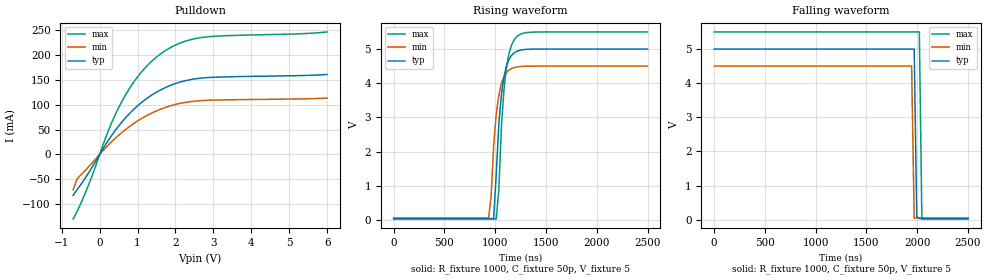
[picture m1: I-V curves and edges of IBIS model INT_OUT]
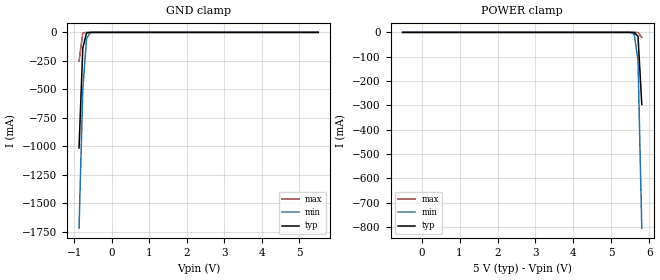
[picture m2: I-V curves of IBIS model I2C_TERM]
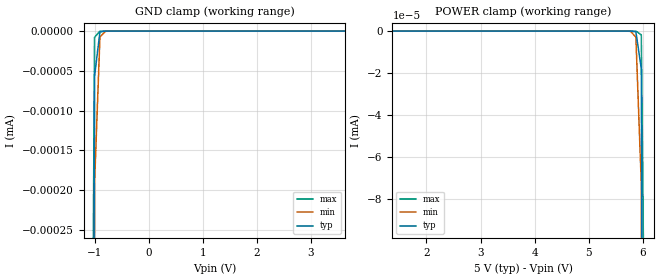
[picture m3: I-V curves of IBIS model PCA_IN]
|   NXP Semiconductors Inc.
|   Specialty Logic Products Group
|   IBIS model of PCA9545B
|   4-Channel I2C switch with
|   interrupt logic and reset
[IBIS Ver]   3.2
[Comment Char]   |_char
|  VDD Typ: 5V, Min: 4.5V, Max: 5.5V
[File name]   pca9545b_5v.ibs
[File Rev]   1.0
[Date]   Dec 05, 2007 9:30:50 AM
[Source]
Generated by Seshadri Venkataramanan with IbisToolKit at Tempe, AZ
[Notes]
[Disclaimer]
(C) Copyright 2007 NXP Semiconductors
All rights reserved
NXP Semiconductors (NXP) does not warrant that this model and any other
accompanying information (Model) accurately or fully represents the
operating characteristics and specifications of the semiconductor
products to which the Model relates.  Moreover, the Model is furnished
on an "as is" and with "all faults" basis, and without support or
warranty of any kind.  NXP disclaims all warranties, whether expressed
or implied or statutory, including without limitation all implied
warranties of non-infringement, merchantability and fitness for any
purpose, and those arising from a course of dealing or usage of trade.
NXP does not convey any license under its or any third party's patents,
copyrights or other intellectual property or proprietary rights.
You and your company assume any and all risks and liability arising out
of the application or use of the Model.
In no event shall NXP be liable for any direct, indirect, special,
consequential or incidental damages, however caused, whether in
warranty, contract or tort (including negligence), strict liability or
other legal theory, including, without limitation, for lost profits,
business interruption, or corruption or loss of data or information,
arising out of or in connection with the use of or the inability to use
the Model, even if NXP has been advised of the possibility of such
damages.
NXP provides the Model as a courtesy to our customers. You and your
company shall not distribute, convey, sell, or give the Model to anyone
else without receiving prior written permission from NXP.
NXP reserves the right to make changes without notice to the Model to
improve reliability, function, or design.
Please be aware that your receipt and subsequent use of the Model shall
serve as acceptance of these terms and conditions.  If you do not
accept these terms, return or destroy the Model immediately.
[Copyright]
2007
[Component]   PCA9545AD
Si_location Pin
Timing_location Pin
[Manufacturer]   NXP Semiconductors
[Package]
|   variable   typ   min   max
R_pkg   5.95E-02   5.36E-02   6.59E-02
L_pkg   4.21E-09   3.07E-09   5.91E-09
C_pkg   0.910E-12   0.758E-12   1.110E-12
|   SO20
[Pin] signal_name   model_name   R_pin   L_pin   C_pin
1   A0   PCA_IN   5.75E-02  5.91E-09  1.050E-12
2   A1   PCA_IN   6.25E-02  4.85E-09  1.040E-12
3   RESETB   PCA_IN   6.59E-02  3.92E-09  0.861E-12
4   INT0B   INT_IN   5.79E-02  3.32E-09  0.803E-12
5   SD0   I2C_TERM   5.36E-02  3.07E-09  0.758E-12
6   SC0   I2C_TERM   5.36E-02  3.07E-09  0.758E-12
7   INT1B   INT_IN   5.79E-02  3.32E-09  0.803E-12
8   SD1   I2C_TERM   6.59E-02  3.92E-09  0.861E-12
9   SC1   I2C_TERM   6.25E-02  4.85E-09  1.040E-12
10   Vss   GND   5.75E-02  5.91E-09  1.110E-12
11   INT2B   INT_IN   5.75E-02  5.91E-09  1.110E-12
12   SD2   I2C_TERM   6.25E-02  4.85E-09  1.040E-12
13   SC2   I2C_TERM   6.59E-02  3.92E-09  0.861E-12
14   INT3B   INT_IN   5.79E-02  3.32E-09  0.803E-12
15   SD3   I2C_TERM   5.36E-02  3.07E-09  0.758E-12
16   SC3   I2C_TERM   5.36E-02  3.07E-09  0.758E-12
17   INTB   INT_OUT   5.79E-02  3.32E-09  0.803E-12
18   SCL   I2C_TERM   6.59E-02  3.92E-09  0.861E-12
19   SDA   I2C_TERM   6.25E-02  4.85E-09  1.040E-12
20   Vdd   POWER   5.75E-02  5.91E-09  1.110E-12
[Component]   PCA9545APW
Si_location Pin
Timing_location Pin
[Manufacturer]   NXP Semiconductors
[Package]
|   variable   typ   min   max
R_pkg   7.24E-02   6.63E-02   8.34E-02
L_pkg   2.47E-09   2.09E-09   3.18E-09
C_pkg   0.341E-12   0.282E-12   0.420E-12
|   TSSOP20
[Pin] signal_name   model_name   R_pin   L_pin   C_pin
1   A0   PCA_IN   6.63E-02  3.18E-09  0.408E-12
2   A1   PCA_IN   6.67E-02  2.55E-09  0.398E-12
3   RESETB   PCA_IN   8.34E-02  2.35E-09  0.317E-12
4   INT0B   INT_IN   7.44E-02  2.16E-09  0.293E-12
5   SD0   I2C_TERM   7.10E-02  2.09E-09  0.282E-12
6   SC0   I2C_TERM   7.10E-02  2.09E-09  0.282E-12
7   INT1B   INT_IN   7.44E-02  2.16E-09  0.293E-12
8   SD1   I2C_TERM   8.34E-02  2.35E-09  0.317E-12
9   SC1   I2C_TERM   6.67E-02  2.55E-09  0.397E-12
10   Vss   GND   6.63E-02  3.18E-09  0.420E-12
11   INT2B   INT_IN   6.63E-02  3.17E-09  0.420E-12
12   SD2   I2C_TERM   6.67E-02  2.55E-09  0.397E-12
13   SC2   I2C_TERM   8.34E-02  2.35E-09  0.317E-12
14   INT3B   INT_IN   7.44E-02  2.16E-09  0.293E-12
15   SD3   I2C_TERM   7.10E-02  2.09E-09  0.282E-12
16   SC3   I2C_TERM   7.10E-02  2.09E-09  0.282E-12
17   INTB   INT_OUT   7.44E-02  2.16E-09  0.293E-12
18   SCL   I2C_TERM   8.34E-02  2.35E-09  0.317E-12
19   SDA   I2C_TERM   6.67E-02  2.55E-09  0.398E-12
20   Vdd   POWER   6.63E-02  3.17E-09  0.420E-12
[Component]   PCA9545ABS
Si_location Pin
Timing_location Pin
[Manufacturer]   NXP Semiconductors
[Package]
|   variable   typ   min   max
R_pkg   0.364   0.215   0.513
L_pkg   1.49E-09   1.04E-09   1.93E-09
C_pkg   0.149E-12   0.124E-12   0.173E-12
|   HVQFN20
[Package Model]   hvqfn20
[Pin] signal_name   model_name
1   RESETB   I2C_TERM
2   INT0B   INT_IN
3   SD0   I2C_TERM
4   SC0   I2C_TERM
5   INT1B   INT_IN
6   SD1   I2C_TERM
7   SC1   I2C_TERM
8   Vss   GND
9   INT2B   INT_IN
10   SD2   I2C_TERM
11   SC2   I2C_TERM
12   INT3B   INT_IN
13   SD3   I2C_TERM
14   SC3   I2C_TERM
15   INTB   INT_OUT
16   SCL   I2C_TERM
17   SDA   I2C_TERM
18   Vdd   POWER
19   A0   PCA_IN
20   A1   PCA_IN
[Series Pin Mapping] pin_2 model_name   function_table_group
18   6   PCA_SW   1
18   9   PCA_SW   2
18   13   PCA_SW   3
18   16   PCA_SW   4
19   5   PCA_SW   1
19   8   PCA_SW   2
19   12   PCA_SW   3
19   15   PCA_SW   4
[Series Switch Groups]
|   Function Group States
|  default
Off 1 2 3 4 /
On 1 /
On 2 /
On 3 /
On 4 /
[Define Package Model]   hvqfn20
[Manufacturer]   Unknown
[OEM]   Unknown
[Description]   none
[Number of Pins]   20
[Pin Numbers]
|   1 = RESETB
1
|   2 = INT0B
2
|   3 = SD0
3
|   4 = SC0
4
|   5 = INT1B
5
|   6 = SD1
6
|   7 = SC1
7
|   8 = VSS
8
|   9 = INT2B
9
|   10 = SD2
10
|   11 = SC2
11
|   12 = INT3B
12
|   13 = SD3
13
|   14 = SC3
14
|   15 = INTB
15
|   16 = SCL
16
|   17 = SDA
17
|   18 = VDD
18
|   19 = A0
19
|   20 = A1
20
[Model Data]
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[End Model Data]
[End Package Model]
[Model]   PCA_SW
Model_type Series_switch
C_comp   0.5p   0.5p   0.5p
[Temperature Range] 27   -40   85
[Voltage Range]   3.3   2.3   5.5
[Pullup Reference]  3.3   2.3   5.5
[Pulldown Reference]0   0   0
[On]
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[Off]
|   variable   R(typ)   R(min)   R(max)
[R Series]   1e06   1e06   1e06
|[End   PCA_SW
| [End   PCA_SW
| Models and submodels in the file (5): INT_OUT (Open_drain), I2C_TERM (Terminator), PCA_IN (Input), INT_IN (Input), PCA_SW (Series_switch)
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[Model]   INT_OUT
Model_type Open_drain
Vref=5
Vmeas=1.65
Rref=1000
Cref=1p
C_comp   2.2p   2p   2.3p
[Model Spec]
Vmeas   1.65   1.485   1.815
[Temperature Range] 27   85   -40
[Voltage Range]   5   4.5   5.5
[Pullup Reference]  5   4.5   5.5
[Pulldown Reference]0   0   0
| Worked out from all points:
|   slope of the pulldown table from 0 to 0.75 V, typ, clamps not added: 9.45 ohm
|   falling waveform, R_fixture 1000, C_fixture 50p, V_fixture 5: 20-80 % time 15.3ns typ, 15.2ns min, 15.1ns max; typ from 5 V to 0.038 V
|   rising waveform, R_fixture 1000, C_fixture 50p, V_fixture 5: 20-80 % time 73.3ns typ, 69.7ns min, 69.8ns max; typ from 0.038 V to 5 V
[Pulldown]
-700mV    -82.55mA   -71.37mA   -130.3mA
-600mV    -71.47mA   -49.68mA   -115.5mA
-300mV    -38.1mA    -25.71mA   -63.01mA
100mV     12.95mA    8.51mA     22.02mA
300mV     36.57mA    24.33mA    61.11mA
600mV     66.6mA     45.04mA    108.9mA
800mV     83.41mA    56.95mA    134.7mA
1.1V      104.4mA    72.13mA    165.9mA
1.6V      129.8mA    90.92mA    202.2mA
2.1V      145.3mA    102.5mA    223.8mA
2.7V      153.9mA    108.5mA    235.7mA
6V        161.1mA    113.4mA    246.9mA
[Falling Waveform]
R_fixture=1000
C_fixture=50p
V_fixture=5
V_fixture_min=4.5
V_fixture_max=5.5
0s        5V         4.5V       5.5V
1.944us   5V         4.5V       5.5V
1.97us    5V         52.35mV    5.5V
1.995us   96.7mV     51.74mV    5.5V
2.02us    37.66mV    51.74mV    5.5V
2.045us   37.66mV    51.74mV    22.54mV
2.5us     37.66mV    51.73mV    24.19mV
[Rising Waveform]
R_fixture=1000
C_fixture=50p
V_fixture=5
V_fixture_min=4.5
V_fixture_max=5.5
0s        37.66mV    51.74mV    24.19mV
934.3ns   37.7mV     51.77mV    24.26mV
959.6ns   37.7mV     676.9mV    24.26mV
984.8ns   37.74mV    2.18V      24.26mV
1.01us    1.341V     3.093V     24.3mV
1.035us   2.781V     3.647V     866.1mV
1.061us   3.655V     3.983V     2.692V
1.111us   4.506V     4.31V      4.47V
1.212us   4.933V     4.474V     5.362V
2.5us     5V         4.5V       5.5V
[Ramp]
R_load=1000
dV/dt_r   1.489E+0/8.641E-10   1.483E+0/1.052E-9   1.493E+0/6.606E-10
dV/dt_f   1.489E+0/3.855E-10   1.483E+0/6.984E-10   1.493E+0/2.039E-10
|[End   INT_OUT
| [End   I2C_TERM
|  [End   I2C_TERM
[Model]   I2C_TERM
Model_type Terminator
C_comp   9.5p   9.5p   9.5p
[Temperature Range] 27   85   -40
[Voltage Range]   5   4.5   5.5
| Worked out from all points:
|   GND clamp passes 1 mA (typ) near -0.59 V on its own axis
[GND Clamp]
|   -6.000000E-1   -1.554225E-1   -1.242642E-1   -2.666059E-1
|   -5.000000E-1   -1.602113E-1   -1.179351E-1   -2.662641E-1
|   -4.000000E-1   -1.574088E-1   -1.099432E-1   -2.800035E-1
-870mV    -1.015A    -1.719A    -253.7mA
-770mV    -138mA     -506.2mA   -5.135mA
-670mV    -5.563mA   -53.39mA   -37.37uA
-570mV    -124.5uA   -3.085mA   -257.8nA
5.5V      942.7pA    1.037nA    987.3pA
[POWER Clamp]
-500mV    942.7pA    1.037nA    987.3pA
5.4V      -174.5nA   -13.1uA    -133.3pA
5.5V      -8.329uA   -332.8uA   -8.003nA
5.6V      -395.8uA   -7.677mA   -1.147uA
5.7V      -15.98mA   -114.2mA   -166.1uA
5.8V      -296.4mA   -804.7mA   -20.01mA
[Model]   PCA_IN
Model_type Input
Vinh=2.1
Vinl=0.9
C_comp   1.73p   1.73p   1.73p
[Temperature Range] 27   85   -40
[Voltage Range]   5   4.5   5.5
[POWER Clamp Reference]5   4.5   5.5
[GND Clamp Reference]0   0   0
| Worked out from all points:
|   GND clamp passes 1 mA (typ) near -1.21 V on its own axis
[GND Clamp]
-3.3V     -35.52A    -34.27A    -37.05A
-1.1V     -2.718uA   -4.916uA   -1.14uA
-1V       -56.9nA    -192.5nA   -7.858nA
-900mV    -1.192nA   -7.538nA   -55.05pA
-800mV    -25.74pA   -295.9pA   -1.173pA
-700mV    -1.222pA   -12.26pA   -702.6fA
3.63V     3.63pA     3.63pA     3.63pA
[POWER Clamp]
1.37V     3.63pA     3.63pA     3.63pA
5.67V     -833.7fA   -5.042pA   -670.6fA
5.77V     -8.589pA   -112.4pA   -853.8fA
5.87V     -374.3pA   -2.852nA   -13.03pA
5.97V     -17.84nA   -72.82nA   -1.766nA
6.07V     -852.2nA   -1.86uA    -256.1nA
8.27V     -34.93A    -33.68A    -36.46A
